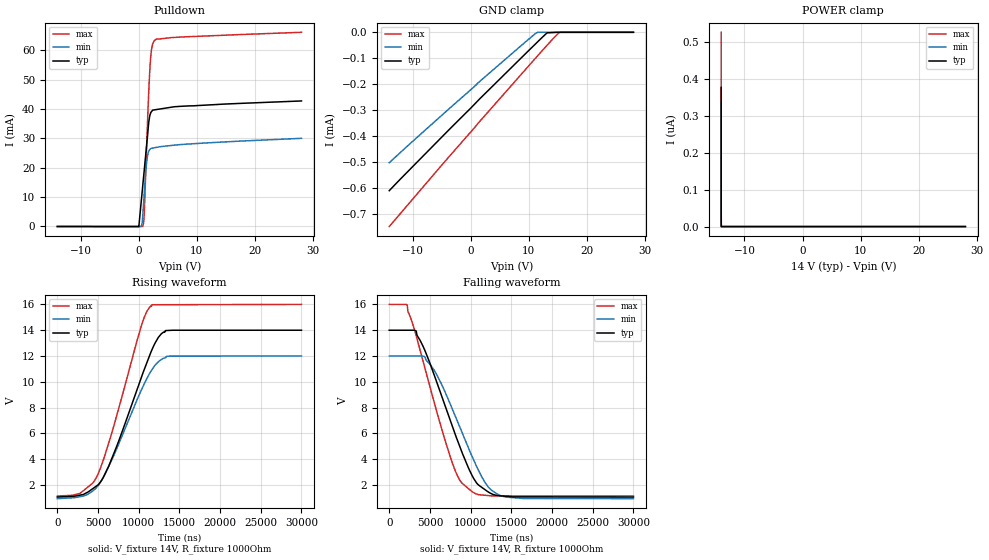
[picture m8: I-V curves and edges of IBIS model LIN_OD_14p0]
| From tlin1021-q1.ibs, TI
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|   LIN_OD_14p0
[Model]   LIN_OD_14p0
Model_type   I/O_open_drain
Polarity   Non-Inverting
Enable   Active-High
Vinl = 5.6
Vinh = 8.4
Vmeas = 7
Vref = 7
Cref = 2pF
Rref = 1000
|   typ   min   max
C_comp   12.71pF   11.59pF   13.31pF
[Voltage Range]   14   12   16
[Temperature Range]   25   165   -55
[Pullup Reference]   14   12   16
[Pulldown Reference]   0   -0   0
[Power Clamp Reference]   14   12   16
[GND Clamp Reference]   0   0   0
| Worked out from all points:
|   slope of the pulldown table from 0 to 2.1 V, typ, clamps not added: 54.1 ohm
|   falling waveform, V_fixture 14V, R_fixture 1000Ohm: 20-80 % time 4.5us typ, 4.52us min, 3.99us max; typ from 14 V to 1.07 V
|   rising waveform, V_fixture 14V, R_fixture 1000Ohm: 20-80 % time 4.52us typ, 4.54us min, 3.98us max; typ from 1.07 V to 14 V
[Pulldown]
|   Voltage   I(typ)   I(min)   I(max)
-14V      -1.801uA   -2.842uA   -1.201uA
25.48mV   -18.3uA    -6.473uA   -6.743uA
508.5mV   9.946mA    254.1uA    2.273uA
723.9mV   14.39mA    4.4mA      250.9uA
923.8mV   18.51mA    10.32mA    3.204mA
1.144V    23.06mA    16.8mA     14.68mA
1.374V    27.8mA     21.9mA     27.56mA
1.677V    34.3mA     25.32mA    43.39mA
1.958V    38.06mA    26.26mA    54.68mA
2.253V    39.19mA    26.62mA    60.76mA
2.805V    39.7mA     26.82mA    63.44mA
28V       42.71mA    29.99mA    66.06mA
[GND Clamp]
|   Voltage   I(typ)   I(min)   I(max)
-14V      -609uA     -501.5uA   -747uA
1.374V    -260.2uA   -192.5uA   -347.3uA
11.3V     -41.54uA   -2.445uA   -95.98uA
13.16V    -2.06uA    0A         -49.37uA
15.2V     0A         0A         -1.688uA
28V       0A         0A         0A
[POWER Clamp]
|   Voltage   I(typ)   I(min)   I(max)
-14V      376.4nA    334.9nA    525.4nA
-14V      0A         0A         149.4nA
-14V      0A         0A         133.4nA
-14V      0A         0A         120.8nA
-14V      0A         0A         105nA
-14V      0A         0A         83.06nA
-14V      0A         0A         63.91nA
-13.99V   0A         0A         46.55nA
-13.99V   0A         0A         25.48nA
-13.97V   0A         0A         0A
28V       0A         0A         0A
[Ramp]
R_load = 1000
|   typ   min   max
dV/dt_r   7.75463/4.50162e-06   6.62965/4.52616e-06   8.90692/3.974e-06
dV/dt_f   7.75468/4.49336e-06   6.6297/4.50769e-06   8.90697/3.98013e-06
[Falling Waveform]
V_fixture = 14V
V_fixture_min = 12V
V_fixture_max = 16V
R_fixture = 1000Ohm
C_fixture = 0F
|   Time   V(typ)   V(min)   V(max)
0s        14V        12V        16V
2.194us   14V        12V        15.96V
3.298us   13.95V     12V        13.6V
5.479us   10.61V     10.94V     8.512V
7.734us   6.596V     7.919V     3.752V
8.679us   4.972V     6.484V     2.369V
10.01us   2.959V     4.465V     1.583V
11.86us   1.605V     2.124V     1.209V
13.75us   1.168V     1.166V     1.166V
30us      1.075V     950.4mV    1.155V
[Rising Waveform]
V_fixture = 14V
V_fixture_min = 12V
V_fixture_max = 16V
R_fixture = 1000Ohm
C_fixture = 0F
|   Time   V(typ)   V(min)   V(max)
0s        1.075V     950.4mV    1.155V
2.753us   1.219V     1.099V     1.354V
4.798us   1.924V     1.799V     2.58V
6.316us   3.467V     3.444V     5.262V
10.35us   10.37V     9.395V     14.39V
10.98us   11.45V     10.23V     15.43V
11.63us   12.48V     10.94V     15.97V
12.43us   13.45V     11.56V     15.97V
13.29us   13.97V     11.86V     15.97V
30us      14V        12V        16V
